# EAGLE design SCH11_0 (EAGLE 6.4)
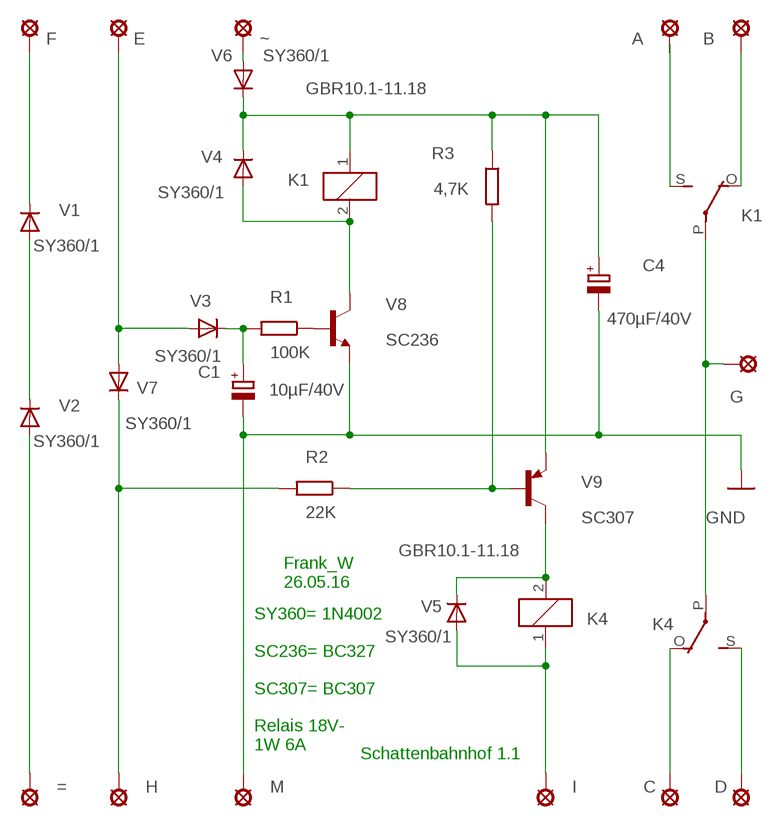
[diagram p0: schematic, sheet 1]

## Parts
=  LSP10  [LSP10]
A  LSP10  [LSP10]
B  LSP10  [LSP10]
C  LSP10  [LSP10]
C1  10µF/40V  CPOL-EUE5-5  [E5-5]
C4  470µF/40V  CPOL-EUE22-9AXIAL  [E22-9]
D  LSP10  [LSP10]
E  LSP10  [LSP10]
F  LSP10  [LSP10]
G  LSP10  [LSP10]
H  LSP10  [LSP10]
I  LSP10  [LSP10]
K1  GBR10.1-11.18  G2R  [G2R]
K4  GBR10.1-11.18  G2R  [G2R]
M  LSP10  [LSP10]
R1  100K  R-EU_0207/12  [0207/12]
R2  22K  R-EU_0207/12  [0207/12]
R3  4,7K  R-EU_0207/12  [0207/12]
V1  SY360/1  1N4004  [DO41-10]
V2  SY360/1  1N4004  [DO41-10]
V3  SY360/1  1N4004  [DO41-10]
V4  SY360/1  1N4004  [DO41-10]
V5  SY360/1  1N4004  [DO41-10]
V6  SY360/1  1N4004  [DO41-10]
V7  SY360/1  1N4004  [DO41-10]
V8  SC236  BC449  [TO92-EBC]
V9  SC307  BC448  [TO92-EBC]
~  LSP10  [LSP10]

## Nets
GND: C1.- C4.- M.MP V8.E
N$1: =.MP V2.A
N$2: V1.A V2.C
N$3: R1.1 V8.B
N$4: F.MP V1.C
N$5: E.MP V3.A V7.A
N$6: C1.+ R1.2 V3.C
N$8: K1.2 V4.A V8.C
N$9: V6.A ~.MP
N$10: C4.+ K1.1 R3.1 V4.C V6.C V9.E
N$11: H.MP R2.2 V7.C
N$12: R2.1 R3.2 V9.B
N$13: K4.2 V5.C V9.C
N$14: G.MP K1.P(2:P) K4.P(2:P)
N$16: B.MP K1.O(2:O)
N$17: A.MP K1.S(2:S)
N$18: C.MP K4.O(2:O)
N$19: D.MP K4.S(2:S)
N$38: I.MP K4.1 V5.A

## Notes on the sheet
- Frank_W
  26.05.16
- SY360= 1N4002
  
  SC236= BC327
  
  SC307= BC307
  
  Relais 18V-
  1W 6A
- Schattenbahnhof 1.1

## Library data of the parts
= A B C D E F G H I M ~ = solpad:LSP10: SOLDER PAD
C1 C4 = rcl:CPOL-EU: POLARIZED CAPACITOR, European symbol
K1 K4 = relay:G2R: RELAY 1 x switch, Omron; OC_FARNELL: 1569185; OC_NEWARK: unknown
R1-R3 = rcl:R-EU_: RESISTOR, European symbol
V1-V7 = diode:1N4004: DIODE
V8 = transistor-npn:BC449*: NPN Transistor
V9 = transistor-pnp:BC448*: PNP Transistror

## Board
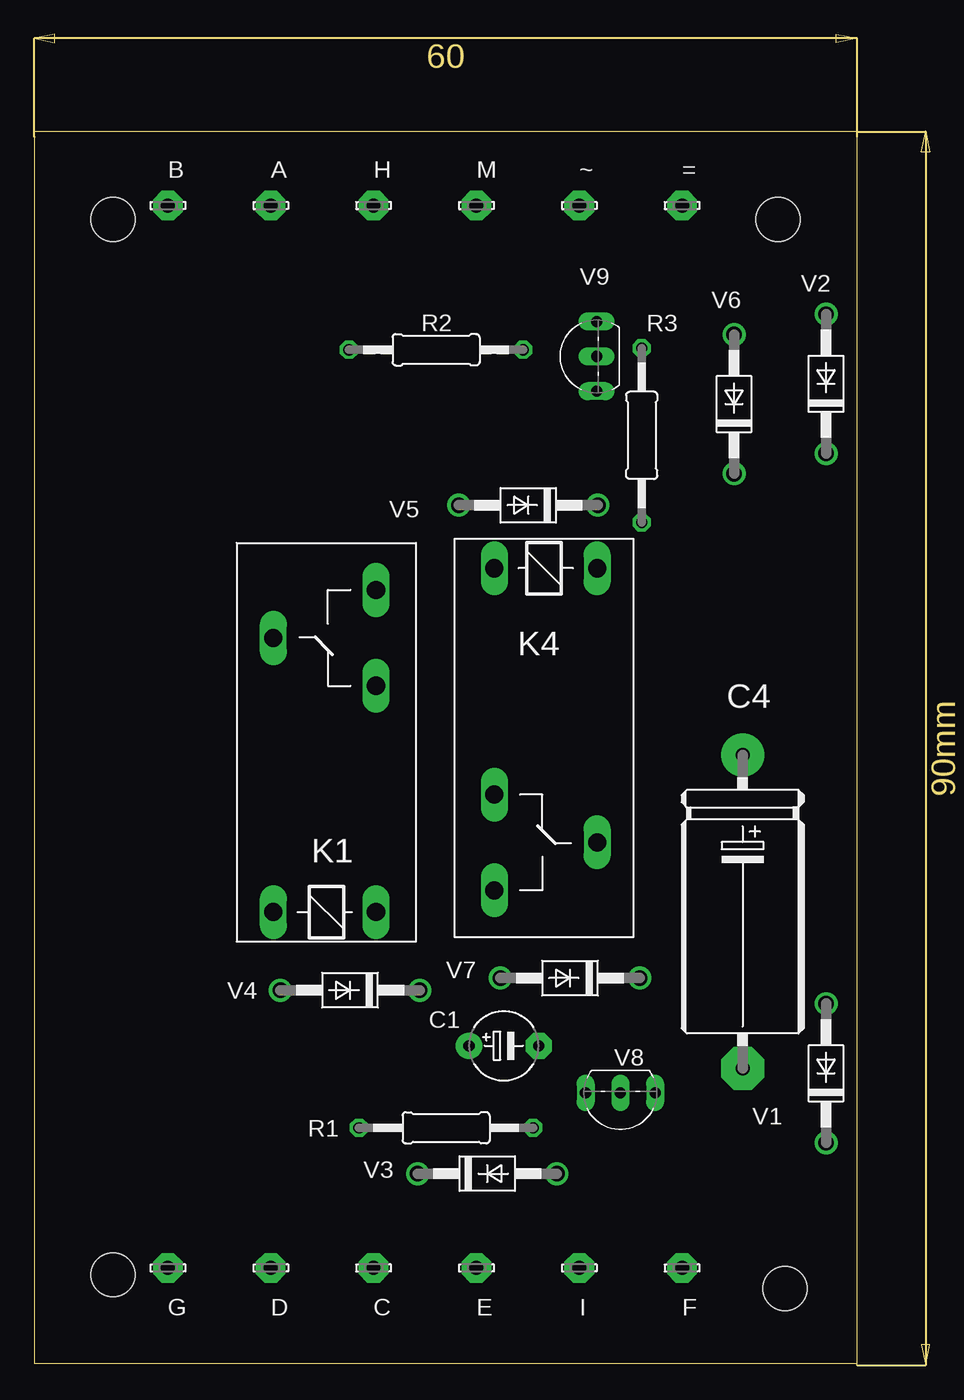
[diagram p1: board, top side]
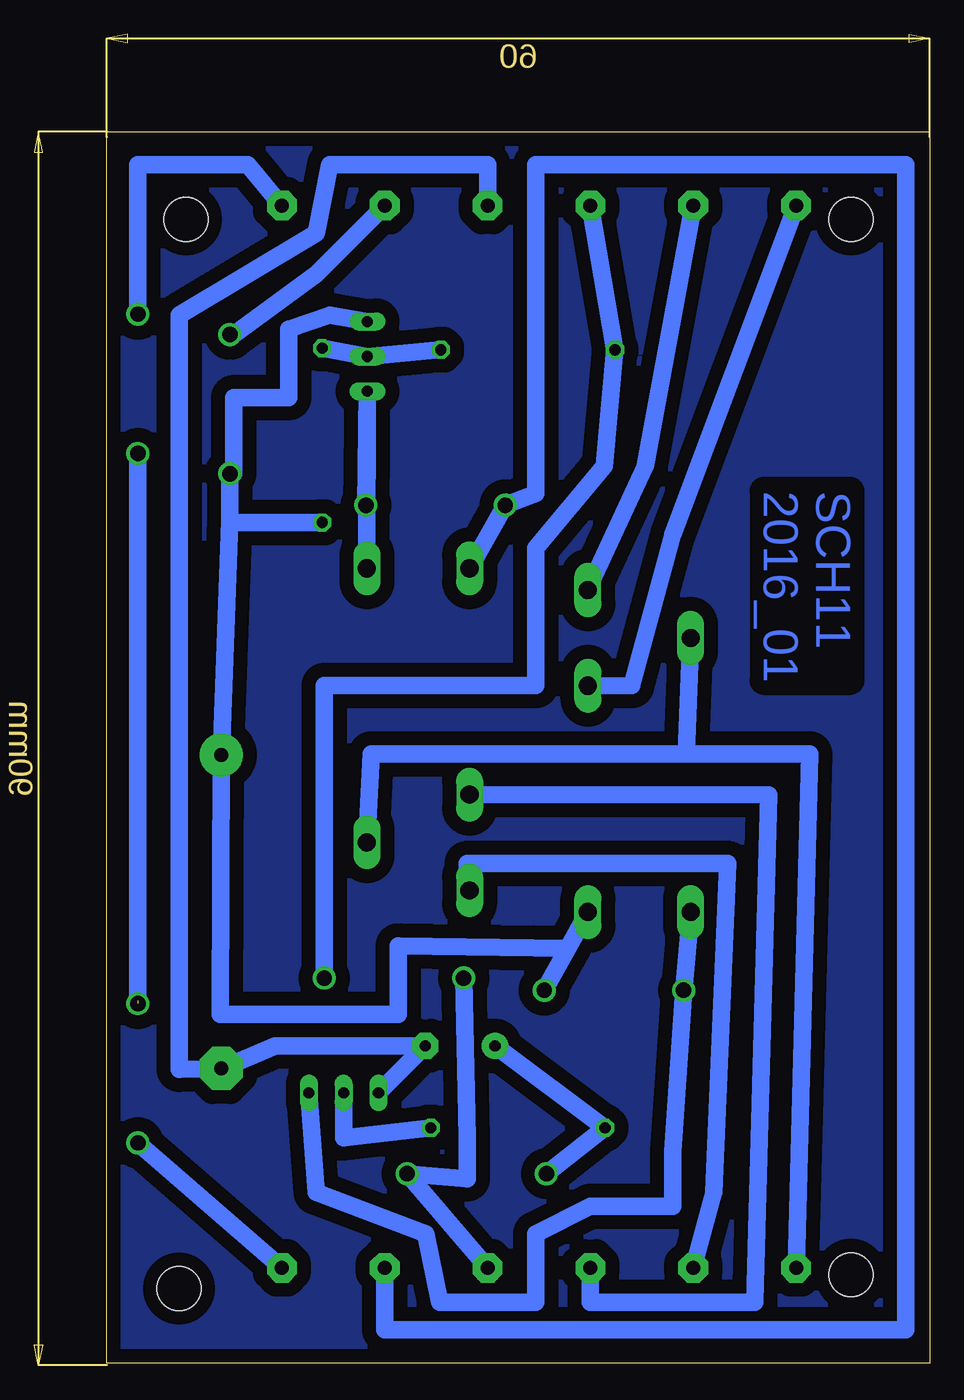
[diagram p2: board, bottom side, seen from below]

Size 65.3 x 97.1 mm. Coordinates in mm from the lower left corner, seen from the top.
Outline: 0,90 0,0.16 60,0.16 60,90 0,90
Copper layers (1*16): Top 0.035mm / dielectric 1.5mm / Bottom 0.035mm
Design rules "default *": minimum track width 20mil, minimum drill 24mil, track to track 8mil, track to pad 8mil, pad to pad 8mil, via to via 8mil, smd to smd 8mil, copper to edge 40mil, drill to drill 8mil, minimum pad ring 10mil, minimum via ring 8mil, stop-mask expansion 4mil, vias tented up to drill 0mil, thermal gap 20mil
Holes 3.2 mm at 54.74,5.6 5.74,6.6 5.74,83.6 54.24,83.6

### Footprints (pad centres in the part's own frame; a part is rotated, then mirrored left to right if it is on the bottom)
LSP10 = drill 1.016 pad 2.159 octagon: MP 0,0
E5-5 = drill 0.813 pad 1.905: + -2.54,0 | drill 0.813 pad 1.905 octagon: - 2.54,0
E22-9 = drill 1.016 pad 3.15: + -11.43,0 | drill 1.016 pad 3.15 octagon: - 11.43,0
G2R = drill 1.321 long: 1 -2.54,-3.683; 2 -2.54,3.81; O 13.97,-3.683; P 17.45,3.81; S 20.955,-3.683
0207/12 = drill 0.813 octagon: 1 -6.35,0; 2 6.35,0
DO41-10 = drill 1.118: A 5.08,0; C -5.08,0
TO92-EBC = drill 0.813 long: B 0,-1.27; C -2.54,-1.27; E 2.54,-1.27

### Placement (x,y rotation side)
=  47.24,84.6 0 top
A  17.24,84.6 0 top
B  9.74,84.6 0 top
C  24.74,7.1 0 top
C1  34.24,23.31 0 top
C4  51.66,33.09 270 top
D  17.24,7.1 0 top
E  32.24,7.1 0 top
F  47.24,7.1 0 top
G  9.74,7.1 0 top
H  24.74,84.6 0 top
I  39.74,7.1 0 top
K1  21.24,35.6 90 top
K4  37.24,55.6 270 top
M  32.24,84.6 0 top
R1  30.03,17.32 180 top
R2  29.3,74.08 180 top
R3  44.3,67.84 90 top
V1  57.74,21.3 90 top
V2  57.74,71.6 90 top
V3  33.03,13.98 0 top
V4  23.03,27.36 180 top
V5  36.03,62.74 180 top
V6  51.03,70.12 90 top
V7  39.07,28.24 180 top
V8  42.74,18.6 180 top
V9  39.74,73.6 90 top
~  39.74,84.6 0 top

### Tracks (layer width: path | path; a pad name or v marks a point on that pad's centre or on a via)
GND
  Bottom 1.27: V8.E C1.- 47.74,23.31 51.74,21.6 C4.- 54.74,21.6 54.74,76.6 44.74,82.6 43.74,87.6 32.24,87.6 M.MP
N$1
  Bottom 1.27: V2.A 57.74,87.6 49.74,87.6 =.MP
N$2  (1 unrouted)
  Bottom 1.27: V2.C 57.74,26.6
N$3
  Bottom 1.27: V8.B 42.74,16.6 R1.1
N$4
  Bottom 1.27: F.MP V1.C
N$5
  Bottom 1.27: E.MP V3.A 33.74,13.6 33.74,16.6 V7.A
N$6
  Bottom 1.27: C1.+ R1.2 V3.C
N$7
  pour Bottom (isolate 1.016): -0.26,89.6 59.74,89.6 59.74,-0.4 -0.26,-0.4 -0.26,88.6
N$8
  Bottom 1.27: K1.2 V4.A 18.74,15.6 18.74,11.6 24.74,11.6 28.74,9.6 28.74,4.6 35.74,4.6 36.74,9.6 44.74,12.6 V8.C
N$9
  Bottom 1.27: V6.A 50.74,75.2 44.74,79.6 ~.MP
N$10
  Bottom 1.27: V9.E 43.74,76.6 46.74,75.6 46.74,70.6 50.74,70.6 50.74,65.04 V6.C 51.03,61.6 | V4.C 26.4,30.41 | 26.4,30.41 K1.1 | 26.4,30.41 38.74,30.6 38.74,25.6 51.74,25.6 C4.+ 51.03,61.6 | R3.1 51.03,61.49 51.03,61.6
N$11
  Bottom 1.27: H.MP R2.2 23.74,65.6 28.74,59.6 28.74,49.6 44.15,49.6 V7.C
N$12
  Bottom 1.27: R2.1 V9.B R3.2
N$13
  Bottom 1.27: V5.C V9.C K4.2
N$14
  Bottom 1.27: 17.74,52.6 K1.P 17.74,44.6 | K4.P 40.74,44.6 17.74,44.6 | 17.74,44.6 8.74,44.6 G.MP
N$16
  Bottom 1.27: K1.O 21.74,49.6 18.74,60.6 B.MP
N$17
  Bottom 1.27: K1.S 20.74,65.6 A.MP
N$18
  Bottom 1.27: K4.O 11.74,41.6 12.74,4.6 24.74,4.6 C.MP
N$19
  Bottom 1.27: D.MP 15.74,12.6 14.74,36.6 33.74,36.6 33.74,34.6 K4.S
N$38
  Bottom 1.27: K4.1 V5.A 28.74,63.6 28.74,87.6 1.74,87.6 1.74,2.6 39.74,2.6 I.MP

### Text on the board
Bottom: SCH11 / 2016_01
